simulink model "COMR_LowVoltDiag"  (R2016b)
settings: Solver=FixedStepDiscrete  StartTime=0.0  StopTime=10.0  FixedStep=1  RelTol=1e-3  EnableMultiTasking=on
undefined symbols (not defined in the file or in its folder): COMR_tiCSCPwrSpy_C, COMR_tiKl30cLowErr_C, COMR_tiKl30HighLowErr_C, COMR_tiKl30OurRang_C, COMR_uCSCVoltHiErr_C, COMR_uCSCVoltLoErr_C, COMR_uKl30cLowErrHeal_C, COMR_uKl30cLowErrHVOn_C, COMR_uKl30cLowErrNoHVOn_C, COMR_uKl30VlotHiErr_C, COMR_uKl30VlotHiHeal_C, COMR_uKl30VoltLoErr_C, COMR_uKl30VoltLoHeal_C, COMR_uKl30VoltOutRngHi_C, COMR_uKl30VoltOutRngLo_C
libraries: simulink x37

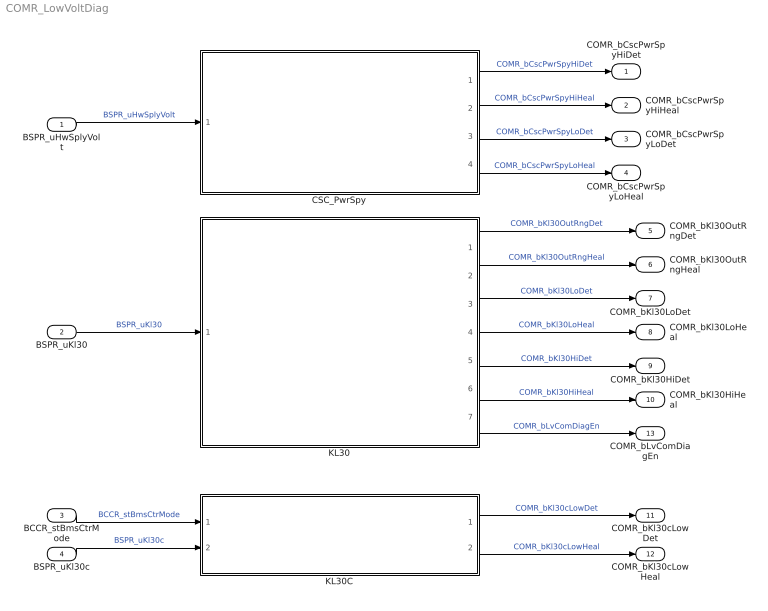
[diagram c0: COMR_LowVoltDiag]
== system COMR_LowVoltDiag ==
  BSPR_uHwSplyVolt : Inport
  BSPR_uKl30 : Inport  Port=2
  BCCR_stBmsCtrMode : Inport  Port=3
  BSPR_uKl30c : Inport  Port=4
  CSC_PwrSpy : Subsystem
  KL30 : Subsystem
  KL30C : Subsystem
  COMR_bCscPwrSpyHiDet : Outport
  COMR_bCscPwrSpyHiHeal : Outport  Port=2
  COMR_bCscPwrSpyLoDet : Outport  Port=3
  COMR_bCscPwrSpyLoHeal : Outport  Port=4
  COMR_bKl30OutRngDet : Outport  Port=5
  COMR_bKl30OutRngHeal : Outport  Port=6
  COMR_bKl30LoDet : Outport  Port=7
  COMR_bKl30LoHeal : Outport  Port=8
  COMR_bKl30HiDet : Outport  Port=9
  COMR_bKl30HiHeal : Outport  Port=10
  COMR_bKl30cLowDet : Outport  Port=11
  COMR_bKl30cLowHeal : Outport  Port=12
  COMR_bLvComDiagEn : Outport  Port=13
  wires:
  BSPR_uHwSplyVolt/1 -> CSC_PwrSpy/1(BSPR_uHwSplyVolt)  "BSPR_uHwSplyVolt"
  BSPR_uKl30/1 -> KL30/1(BSPR_uKl30)  "BSPR_uKl30"
  BCCR_stBmsCtrMode/1 -> KL30C/1(BCCR_stBmsCtrMode)  "BCCR_stBmsCtrMode"
  BSPR_uKl30c/1 -> KL30C/2(BSPR_uKl30c)  "BSPR_uKl30c"
  CSC_PwrSpy/4(COMR_bCscPwrSpyLoHeal) -> COMR_bCscPwrSpyLoHeal/1  "COMR_bCscPwrSpyLoHeal"
  CSC_PwrSpy/1(COMR_bCscPwrSpyHiDet) -> COMR_bCscPwrSpyHiDet/1  "COMR_bCscPwrSpyHiDet"
  CSC_PwrSpy/2(COMR_bCscPwrSpyHiHeal) -> COMR_bCscPwrSpyHiHeal/1  "COMR_bCscPwrSpyHiHeal"
  CSC_PwrSpy/3(COMR_bCscPwrSpyLoDet) -> COMR_bCscPwrSpyLoDet/1  "COMR_bCscPwrSpyLoDet"
  KL30/1(COMR_bKl30OutRngDet) -> COMR_bKl30OutRngDet/1  "COMR_bKl30OutRngDet"
  KL30/2(COMR_bKl30OutRngHeal) -> COMR_bKl30OutRngHeal/1  "COMR_bKl30OutRngHeal"
  KL30/3(COMR_bKl30LoDet) -> COMR_bKl30LoDet/1  "COMR_bKl30LoDet"
  KL30/5(COMR_bKl30HiDet) -> COMR_bKl30HiDet/1  "COMR_bKl30HiDet"
  KL30/4(COMR_bKl30LoHeal) -> COMR_bKl30LoHeal/1  "COMR_bKl30LoHeal"
  KL30/6(COMR_bKl30HiHeal) -> COMR_bKl30HiHeal/1  "COMR_bKl30HiHeal"
  KL30C/1(COMR_bKl30cLowDet) -> COMR_bKl30cLowDet/1  "COMR_bKl30cLowDet"
  KL30C/2(COMR_bKl30cLowHeal) -> COMR_bKl30cLowHeal/1  "COMR_bKl30cLowHeal"
  KL30/7(COMR_bLvComDiagEn) -> COMR_bLvComDiagEn/1  "COMR_bLvComDiagEn"

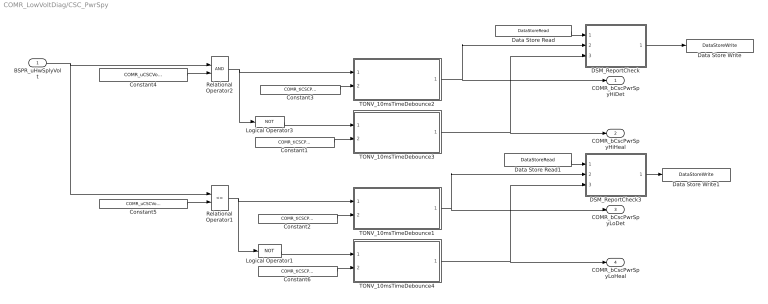
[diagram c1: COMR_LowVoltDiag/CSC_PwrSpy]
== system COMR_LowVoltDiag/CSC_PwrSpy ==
  BSPR_uHwSplyVolt : Inport
  Constant{1..3,6} (4 alike) : Constant  Value=COMR_tiCSCPwrSpy_C
  Constant4 : Constant  Value=COMR_uCSCVoltHiErr_C
  Constant5 : Constant  Value=COMR_uCSCVoltLoErr_C
  DSM_ReportCheck : Subsystem  TreatAsAtomicUnit=on  RTWFcnName=DSM_ReportCheck  RTWFileName=SrvLib
  DSM_ReportCheck3 : Subsystem  TreatAsAtomicUnit=on  RTWFcnName=DSM_ReportCheck  RTWFileName=SrvLib
  Data Store Read : DataStoreRead  DataStoreName=DFC_CSCPwrSpyHiErr
  Data Store Read1 : DataStoreRead  DataStoreName=DFC_CSCPwrSpyLoErr
  Data Store Write : DataStoreWrite  DataStoreName=DFC_CSCPwrSpyHiErr
  Data Store Write1 : DataStoreWrite  DataStoreName=DFC_CSCPwrSpyLoErr
  Logical Operator1 : Logic  Operator=NOT  AllPortsSameDT=off  OutDataTypeStr=boolean
  Logical Operator3 : Logic  Operator=NOT  AllPortsSameDT=off  OutDataTypeStr=boolean
  Relational Operator1 : RelationalOperator  Operator=<=  OutDataTypeStr=boolean  RndMeth=Simplest
  Relational Operator2 : RelationalOperator  OutDataTypeStr=boolean  RndMeth=Simplest
  TONV_10msTimeDebounce1 : Subsystem  TreatAsAtomicUnit=on  RTWFcnName=TONV_10msTimeDebounce  RTWFileName=SrvLib
  TONV_10msTimeDebounce2 : Subsystem  TreatAsAtomicUnit=on  RTWFcnName=TONV_10msTimeDebounce  RTWFileName=SrvLib
  TONV_10msTimeDebounce3 : Subsystem  TreatAsAtomicUnit=on  RTWFcnName=TONV_10msTimeDebounce  RTWFileName=SrvLib
  TONV_10msTimeDebounce4 : Subsystem  TreatAsAtomicUnit=on  RTWFcnName=TONV_10msTimeDebounce  RTWFileName=SrvLib
  COMR_bCscPwrSpyHiDet : Outport
  COMR_bCscPwrSpyHiHeal : Outport  Port=2
  COMR_bCscPwrSpyLoDet : Outport  Port=3
  COMR_bCscPwrSpyLoHeal : Outport  Port=4
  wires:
  Constant4/1 -> Relational Operator2/2
  BSPR_uHwSplyVolt/1 -> Relational Operator2/1, Relational Operator1/1
  TONV_10msTimeDebounce2/1(y) -> DSM_ReportCheck/2(Err), COMR_bCscPwrSpyHiDet/1
  Relational Operator2/1 -> TONV_10msTimeDebounce2/1(u), Logical Operator3/1
  DSM_ReportCheck/1(Dfc_id) -> Data Store Write/1
  Constant3/1 -> TONV_10msTimeDebounce2/2(T)
  Constant2/1 -> TONV_10msTimeDebounce1/2(T)
  Relational Operator1/1 -> Logical Operator1/1, TONV_10msTimeDebounce1/1(u)
  TONV_10msTimeDebounce1/1(y) -> DSM_ReportCheck3/2(Err), COMR_bCscPwrSpyLoDet/1
  DSM_ReportCheck3/1(Dfc_id) -> Data Store Write1/1
  Constant5/1 -> Relational Operator1/2
  Logical Operator3/1 -> TONV_10msTimeDebounce3/1(u)
  Constant1/1 -> TONV_10msTimeDebounce3/2(T)
  TONV_10msTimeDebounce3/1(y) -> DSM_ReportCheck/3(Heal), COMR_bCscPwrSpyHiHeal/1
  Data Store Read/1 -> DSM_ReportCheck/1(Dfc_id_nv)
  Logical Operator1/1 -> TONV_10msTimeDebounce4/1(u)
  Constant6/1 -> TONV_10msTimeDebounce4/2(T)
  TONV_10msTimeDebounce4/1(y) -> DSM_ReportCheck3/3(Heal), COMR_bCscPwrSpyLoHeal/1
  Data Store Read1/1 -> DSM_ReportCheck3/1(Dfc_id_nv)

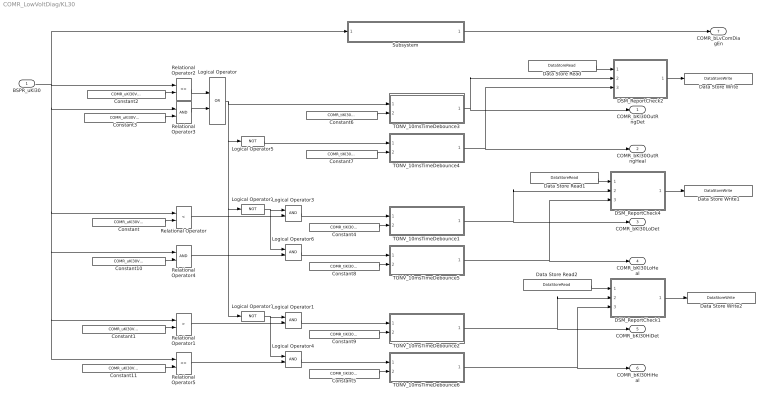
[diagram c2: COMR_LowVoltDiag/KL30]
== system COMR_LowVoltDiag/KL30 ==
  BSPR_uKl30 : Inport
  Constant : Constant  Value=COMR_uKl30VoltLoErr_C
  Constant1 : Constant  Value=COMR_uKl30VlotHiErr_C
  Constant10 : Constant  Value=COMR_uKl30VoltLoHeal_C
  Constant11 : Constant  Value=COMR_uKl30VlotHiHeal_C
  Constant2 : Constant  Value=COMR_uKl30VoltOutRngLo_C
  Constant3 : Constant  Value=COMR_uKl30VoltOutRngHi_C
  Constant{4..5,8..9} (4 alike) : Constant  Value=COMR_tiKl30HighLowErr_C
  Constant6 : Constant  Value=COMR_tiKl30OurRang_C
  Constant7 : Constant  Value=COMR_tiKl30OurRang_C
  DSM_ReportCheck1 : Subsystem  TreatAsAtomicUnit=on  RTWFcnName=DSM_ReportCheck  RTWFileName=SrvLib
  DSM_ReportCheck2 : Subsystem  TreatAsAtomicUnit=on  RTWFcnName=DSM_ReportCheck  RTWFileName=SrvLib
  DSM_ReportCheck4 : Subsystem  TreatAsAtomicUnit=on  RTWFcnName=DSM_ReportCheck  RTWFileName=SrvLib
  Data Store Read : DataStoreRead  DataStoreName=DFC_Kl30OutRngErr
  Data Store Read1 : DataStoreRead  DataStoreName=DFC_Kl30VoltLoErr
  Data Store Read2 : DataStoreRead  DataStoreName=DFC_Kl30VoltHiErr
  Data Store Write : DataStoreWrite  DataStoreName=DFC_Kl30OutRngErr
  Data Store Write1 : DataStoreWrite  DataStoreName=DFC_Kl30VoltLoErr
  Data Store Write2 : DataStoreWrite  DataStoreName=DFC_Kl30VoltHiErr
  Logical Operator : Logic  Operator=OR  AllPortsSameDT=off  OutDataTypeStr=boolean
  Logical Operator{1,3..4,6} (4 alike) : Logic  AllPortsSameDT=off  OutDataTypeStr=boolean
  Logical Operator2 : Logic  Operator=NOT  AllPortsSameDT=off  OutDataTypeStr=boolean
  Logical Operator5 : Logic  Operator=NOT  AllPortsSameDT=off  OutDataTypeStr=boolean
  Logical Operator7 : Logic  Operator=NOT  AllPortsSameDT=off  OutDataTypeStr=boolean
  Relational Operator : RelationalOperator  Operator=<  OutDataTypeStr=boolean  RndMeth=Simplest
  Relational Operator1 : RelationalOperator  Operator=>  OutDataTypeStr=boolean  RndMeth=Simplest
  Relational Operator2 : RelationalOperator  Operator=<=  OutDataTypeStr=boolean  RndMeth=Simplest
  Relational Operator3 : RelationalOperator  OutDataTypeStr=boolean  RndMeth=Simplest
  Relational Operator4 : RelationalOperator  OutDataTypeStr=boolean  RndMeth=Simplest
  Relational Operator5 : RelationalOperator  Operator=<=  OutDataTypeStr=boolean  RndMeth=Simplest
  Subsystem : Subsystem
  TONV_10msTimeDebounce1 : Subsystem  TreatAsAtomicUnit=on  RTWFcnName=TONV_10msTimeDebounce  RTWFileName=SrvLib
  TONV_10msTimeDebounce2 : Subsystem  TreatAsAtomicUnit=on  RTWFcnName=TONV_10msTimeDebounce  RTWFileName=SrvLib
  TONV_10msTimeDebounce3 : Subsystem  TreatAsAtomicUnit=on  RTWFcnName=TONV_10msTimeDebounce  RTWFileName=SrvLib
  TONV_10msTimeDebounce4 : Subsystem  TreatAsAtomicUnit=on  RTWFcnName=TONV_10msTimeDebounce  RTWFileName=SrvLib
  TONV_10msTimeDebounce5 : Subsystem  TreatAsAtomicUnit=on  RTWFcnName=TONV_10msTimeDebounce  RTWFileName=SrvLib
  TONV_10msTimeDebounce6 : Subsystem  TreatAsAtomicUnit=on  RTWFcnName=TONV_10msTimeDebounce  RTWFileName=SrvLib
  COMR_bKl30OutRngDet : Outport
  COMR_bKl30OutRngHeal : Outport  Port=2
  COMR_bKl30LoDet : Outport  Port=3
  COMR_bKl30LoHeal : Outport  Port=4
  COMR_bKl30HiDet : Outport  Port=5
  COMR_bKl30HiHeal : Outport  Port=6
  COMR_bLvComDiagEn : Outport  Port=7
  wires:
  Constant5/1 -> TONV_10msTimeDebounce6/2(T)
  TONV_10msTimeDebounce6/1(y) -> COMR_bKl30HiHeal/1, DSM_ReportCheck1/3(Heal)
  Data Store Read1/1 -> DSM_ReportCheck4/1(Dfc_id_nv)
  Data Store Read2/1 -> DSM_ReportCheck1/1(Dfc_id_nv)
  Logical Operator3/1 -> TONV_10msTimeDebounce1/1(u)
  Constant9/1 -> TONV_10msTimeDebounce2/2(T)
  Constant4/1 -> TONV_10msTimeDebounce1/2(T)
  Relational Operator3/1 -> Logical Operator/2
  Relational Operator2/1 -> Logical Operator/1
  TONV_10msTimeDebounce1/1(y) -> DSM_ReportCheck4/2(Err), COMR_bKl30LoDet/1
  Constant7/1 -> TONV_10msTimeDebounce4/2(T)
  Data Store Read/1 -> DSM_ReportCheck2/1(Dfc_id_nv)
  TONV_10msTimeDebounce2/1(y) -> DSM_ReportCheck1/2(Err), COMR_bKl30HiDet/1
  DSM_ReportCheck1/1(Dfc_id) -> Data Store Write2/1
  TONV_10msTimeDebounce3/1(y) -> COMR_bKl30OutRngDet/1, DSM_ReportCheck2/2(Err)
  DSM_ReportCheck2/1(Dfc_id) -> Data Store Write/1
  Constant6/1 -> TONV_10msTimeDebounce3/2(T)
  Logical Operator5/1 -> TONV_10msTimeDebounce4/1(u)
  DSM_ReportCheck4/1(Dfc_id) -> Data Store Write1/1
  TONV_10msTimeDebounce4/1(y) -> COMR_bKl30OutRngHeal/1, DSM_ReportCheck2/3(Heal)
  Logical Operator/1 -> Logical Operator7/1, Logical Operator2/1, Logical Operator5/1, TONV_10msTimeDebounce3/1(u)
  Logical Operator1/1 -> TONV_10msTimeDebounce2/1(u)
  Constant3/1 -> Relational Operator3/2
  Constant2/1 -> Relational Operator2/2
  TONV_10msTimeDebounce5/1(y) -> COMR_bKl30LoHeal/1, DSM_ReportCheck4/3(Heal)
  Constant8/1 -> TONV_10msTimeDebounce5/2(T)
  Relational Operator4/1 -> Logical Operator6/2
  Relational Operator1/1 -> Logical Operator1/2
  Constant1/1 -> Relational Operator1/2
  Constant/1 -> Relational Operator/2
  BSPR_uKl30/1 -> Relational Operator2/1, Relational Operator3/1, Relational Operator/1, Relational Operator4/1, Relational Operator5/1, Relational Operator1/1, Subsystem/1(BSPR_uKl30)
  Relational Operator/1 -> Logical Operator3/2
  Logical Operator2/1 -> Logical Operator6/1, Logical Operator3/1
  Logical Operator7/1 -> Logical Operator4/1, Logical Operator1/1
  Subsystem/1(COMR_bLvComDiagEn) -> COMR_bLvComDiagEn/1
  Constant10/1 -> Relational Operator4/2
  Constant11/1 -> Relational Operator5/2
  Relational Operator5/1 -> Logical Operator4/2
  Logical Operator4/1 -> TONV_10msTimeDebounce6/1(u)
  Logical Operator6/1 -> TONV_10msTimeDebounce5/1(u)

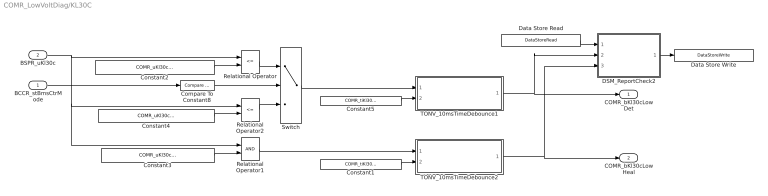
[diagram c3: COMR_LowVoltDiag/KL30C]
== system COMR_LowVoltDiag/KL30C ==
  BCCR_stBmsCtrMode : Inport
  BSPR_uKl30c : Inport  Port=2
  Compare To Constant8 : simulink/Logic and Bit Operations/Compare To Constant  relop===  const=4  OutDataTypeStr=boolean
  Constant1 : Constant  Value=COMR_tiKl30cLowErr_C  OutDataTypeStr=single
  Constant2 : Constant  Value=COMR_uKl30cLowErrHVOn_C  OutDataTypeStr=single
  Constant3 : Constant  Value=COMR_uKl30cLowErrHeal_C  OutDataTypeStr=single
  Constant4 : Constant  Value=COMR_uKl30cLowErrNoHVOn_C  OutDataTypeStr=single
  Constant5 : Constant  Value=COMR_tiKl30cLowErr_C  OutDataTypeStr=single
  DSM_ReportCheck2 : Subsystem  TreatAsAtomicUnit=on  RTWFcnName=DSM_ReportCheck  RTWFileName=SrvLib
  Data Store Read : DataStoreRead  DataStoreName=DFC_Kl30cVoltLoErr
  Data Store Write : DataStoreWrite  DataStoreName=DFC_Kl30cVoltLoErr
  Relational Operator : RelationalOperator  Operator=<=  OutDataTypeStr=boolean  RndMeth=Simplest
  Relational Operator1 : RelationalOperator  OutDataTypeStr=boolean  RndMeth=Simplest
  Relational Operator2 : RelationalOperator  Operator=<=  OutDataTypeStr=boolean  RndMeth=Simplest
  Switch : Switch  Criteria=u2 > Threshold
  TONV_10msTimeDebounce1 : Subsystem  TreatAsAtomicUnit=on  RTWFcnName=TONV_10msTimeDebounce  RTWFileName=SrvLib
  TONV_10msTimeDebounce2 : Subsystem  TreatAsAtomicUnit=on  RTWFcnName=TONV_10msTimeDebounce  RTWFileName=SrvLib
  COMR_bKl30cLowDet : Outport
  COMR_bKl30cLowHeal : Outport  Port=2
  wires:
  Constant1/1 -> TONV_10msTimeDebounce2/2(T)
  Data Store Read/1 -> DSM_ReportCheck2/1(Dfc_id_nv)
  Constant2/1 -> Relational Operator/2
  BSPR_uKl30c/1 -> Relational Operator/1, Relational Operator2/1, Relational Operator1/1
  Relational Operator/1 -> Switch/1
  Constant5/1 -> TONV_10msTimeDebounce1/2(T)
  Relational Operator2/1 -> Switch/3
  TONV_10msTimeDebounce2/1(y) -> COMR_bKl30cLowHeal/1, DSM_ReportCheck2/3(Heal)
  TONV_10msTimeDebounce1/1(y) -> DSM_ReportCheck2/2(Err), COMR_bKl30cLowDet/1
  Compare To Constant8/1 -> Switch/2
  Constant4/1 -> Relational Operator2/2
  BCCR_stBmsCtrMode/1 -> Compare To Constant8/1
  DSM_ReportCheck2/1(Dfc_id) -> Data Store Write/1
  Switch/1 -> TONV_10msTimeDebounce1/1(u)
  Relational Operator1/1 -> TONV_10msTimeDebounce2/1(u)
  Constant3/1 -> Relational Operator1/2

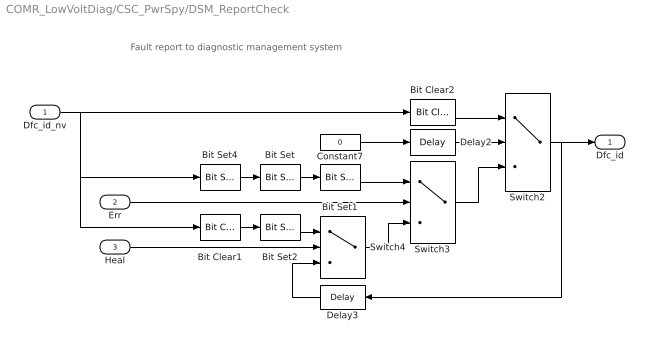
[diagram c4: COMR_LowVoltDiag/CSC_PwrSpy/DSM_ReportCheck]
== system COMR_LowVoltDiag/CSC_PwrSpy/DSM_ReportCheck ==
  note: Fault report to diagnostic management system
  Dfc_id_nv : Inport  OutDataTypeStr=uint8
  Err : Inport  Port=2
  Heal : Inport  Port=3
  Bit Clear1 : simulink/Logic and Bit Operations/Bit Clear  iBit=4
  Bit Clear2 : simulink/Logic and Bit Operations/Bit Clear  iBit=3
  Bit Set : simulink/Logic and Bit Operations/Bit Set  iBit=4
  Bit Set1 : simulink/Logic and Bit Operations/Bit Set  iBit=3
  Bit Set2 : simulink/Logic and Bit Operations/Bit Set  iBit=3
  Bit Set4 : simulink/Logic and Bit Operations/Bit Set  iBit=7
  Constant7 : Constant  Value=0  OutDataTypeStr=boolean
  Delay2 : Delay  DelayLength=1  InitialCondition=1
  Delay3 : Delay  DelayLength=1  InitialCondition=0
  Switch2 : Switch  Criteria=u2 ~= 0
  Switch3 : Switch  Criteria=u2 ~= 0
  Switch4 : Switch  Criteria=u2 ~= 0
  Dfc_id : Outport  OutDataTypeStr=uint8
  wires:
  Dfc_id_nv/1 -> Bit Clear2/1, Bit Set4/1, Bit Clear1/1
  Bit Set4/1 -> Bit Set/1
  Constant7/1 -> Delay2/1
  Delay2/1 -> Switch2/2
  Switch3/1 -> Switch2/3
  Bit Clear2/1 -> Switch2/1
  Switch2/1 -> Delay3/1, Dfc_id/1
  Bit Set1/1 -> Switch3/1
  Bit Set/1 -> Bit Set1/1
  Switch4/1 -> Switch3/3
  Err/1 -> Switch3/2
  Bit Set2/1 -> Switch4/1
  Bit Clear1/1 -> Bit Set2/1
  Delay3/1 -> Switch4/3
  Heal/1 -> Switch4/2

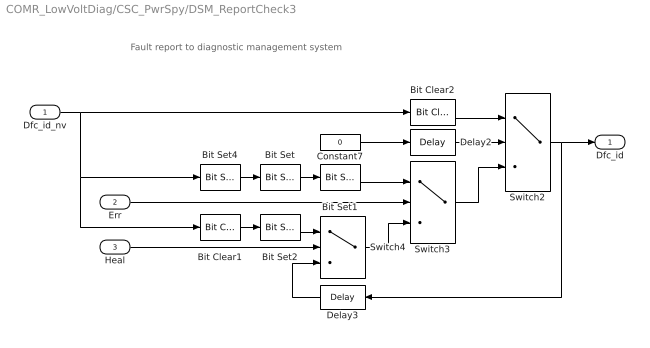
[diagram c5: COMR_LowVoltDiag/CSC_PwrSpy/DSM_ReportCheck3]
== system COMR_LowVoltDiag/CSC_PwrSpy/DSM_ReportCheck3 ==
  note: Fault report to diagnostic management system
  Dfc_id_nv : Inport  OutDataTypeStr=uint8
  Err : Inport  Port=2
  Heal : Inport  Port=3
  Bit Clear1 : simulink/Logic and Bit Operations/Bit Clear  iBit=4
  Bit Clear2 : simulink/Logic and Bit Operations/Bit Clear  iBit=3
  Bit Set : simulink/Logic and Bit Operations/Bit Set  iBit=4
  Bit Set1 : simulink/Logic and Bit Operations/Bit Set  iBit=3
  Bit Set2 : simulink/Logic and Bit Operations/Bit Set  iBit=3
  Bit Set4 : simulink/Logic and Bit Operations/Bit Set  iBit=7
  Constant7 : Constant  Value=0  OutDataTypeStr=boolean
  Delay2 : Delay  DelayLength=1  InitialCondition=1
  Delay3 : Delay  DelayLength=1  InitialCondition=0
  Switch2 : Switch  Criteria=u2 ~= 0
  Switch3 : Switch  Criteria=u2 ~= 0
  Switch4 : Switch  Criteria=u2 ~= 0
  Dfc_id : Outport  OutDataTypeStr=uint8
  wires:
  Dfc_id_nv/1 -> Bit Clear2/1, Bit Set4/1, Bit Clear1/1
  Bit Set4/1 -> Bit Set/1
  Constant7/1 -> Delay2/1
  Delay2/1 -> Switch2/2
  Switch3/1 -> Switch2/3
  Bit Clear2/1 -> Switch2/1
  Switch2/1 -> Delay3/1, Dfc_id/1
  Bit Set1/1 -> Switch3/1
  Bit Set/1 -> Bit Set1/1
  Switch4/1 -> Switch3/3
  Err/1 -> Switch3/2
  Bit Set2/1 -> Switch4/1
  Bit Clear1/1 -> Bit Set2/1
  Delay3/1 -> Switch4/3
  Heal/1 -> Switch4/2

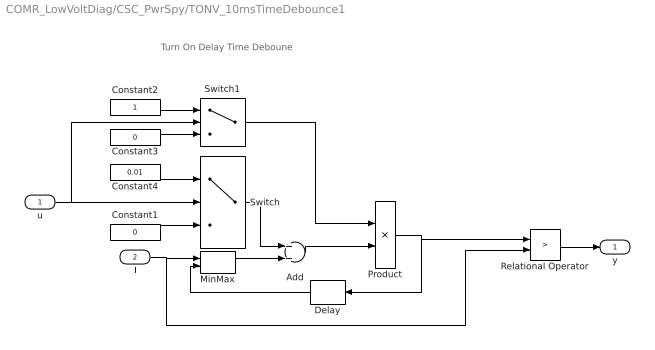
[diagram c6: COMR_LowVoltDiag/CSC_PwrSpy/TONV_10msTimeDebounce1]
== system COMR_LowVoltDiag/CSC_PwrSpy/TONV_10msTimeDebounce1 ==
  note: Turn On Delay Time Deboune
  u : Inport
  T : Inport  Port=2
  Add : Sum
  Constant1 : Constant  Value=0  OutDataTypeStr=single
  Constant2 : Constant  OutDataTypeStr=uint8
  Constant3 : Constant  Value=0  OutDataTypeStr=uint8
  Constant4 : Constant  Value=0.01  OutDataTypeStr=single
  Delay : Delay  DelayLength=1  InitialCondition=0
  MinMax : MinMax  Inputs=2
  Product : Product  OutMin=[0]  OutMax=[65535]  OutDataTypeStr=single
  Relational Operator : RelationalOperator  Operator=>  OutDataTypeStr=boolean  RndMeth=Simplest
  Switch : Switch  Criteria=u2 ~= 0
  Switch1 : Switch  Criteria=u2 ~= 0
  y : Outport
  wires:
  MinMax/1 -> Add/2
  T/1 -> Relational Operator/2, MinMax/1
  Relational Operator/1 -> y/1
  Delay/1 -> MinMax/2
  Switch/1 -> Add/1
  Product/1 -> Delay/1, Relational Operator/1
  Add/1 -> Product/2
  Constant1/1 -> Switch/3
  Constant4/1 -> Switch/1
  u/1 -> Switch/2, Switch1/2
  Constant2/1 -> Switch1/1
  Constant3/1 -> Switch1/3
  Switch1/1 -> Product/1

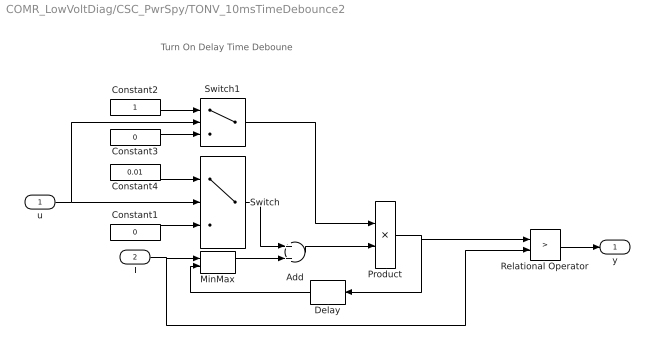
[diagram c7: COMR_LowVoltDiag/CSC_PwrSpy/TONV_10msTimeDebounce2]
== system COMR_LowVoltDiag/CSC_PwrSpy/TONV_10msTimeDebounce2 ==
  note: Turn On Delay Time Deboune
  u : Inport
  T : Inport  Port=2
  Add : Sum
  Constant1 : Constant  Value=0  OutDataTypeStr=single
  Constant2 : Constant  OutDataTypeStr=uint8
  Constant3 : Constant  Value=0  OutDataTypeStr=uint8
  Constant4 : Constant  Value=0.01  OutDataTypeStr=single
  Delay : Delay  DelayLength=1  InitialCondition=0
  MinMax : MinMax  Inputs=2
  Product : Product  OutMin=[0]  OutMax=[65535]  OutDataTypeStr=single
  Relational Operator : RelationalOperator  Operator=>  OutDataTypeStr=boolean  RndMeth=Simplest
  Switch : Switch  Criteria=u2 ~= 0
  Switch1 : Switch  Criteria=u2 ~= 0
  y : Outport
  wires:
  MinMax/1 -> Add/2
  T/1 -> Relational Operator/2, MinMax/1
  Relational Operator/1 -> y/1
  Delay/1 -> MinMax/2
  Switch/1 -> Add/1
  Product/1 -> Delay/1, Relational Operator/1
  Add/1 -> Product/2
  Constant1/1 -> Switch/3
  Constant4/1 -> Switch/1
  u/1 -> Switch/2, Switch1/2
  Constant2/1 -> Switch1/1
  Constant3/1 -> Switch1/3
  Switch1/1 -> Product/1

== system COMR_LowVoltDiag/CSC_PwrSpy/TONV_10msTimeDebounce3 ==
  note: Turn On Delay Time Deboune
  u : Inport
  T : Inport  Port=2
  Add : Sum
  Constant1 : Constant  Value=0  OutDataTypeStr=single
  Constant2 : Constant  OutDataTypeStr=uint8
  Constant3 : Constant  Value=0  OutDataTypeStr=uint8
  Constant4 : Constant  Value=0.01  OutDataTypeStr=single
  Delay : Delay  DelayLength=1  InitialCondition=0
  MinMax : MinMax  Inputs=2
  Product : Product  OutMin=[0]  OutMax=[65535]  OutDataTypeStr=single
  Relational Operator : RelationalOperator  Operator=>  OutDataTypeStr=boolean  RndMeth=Simplest
  Switch : Switch  Criteria=u2 ~= 0
  Switch1 : Switch  Criteria=u2 ~= 0
  y : Outport
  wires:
  MinMax/1 -> Add/2
  T/1 -> Relational Operator/2, MinMax/1
  Relational Operator/1 -> y/1
  Delay/1 -> MinMax/2
  Switch/1 -> Add/1
  Product/1 -> Delay/1, Relational Operator/1
  Add/1 -> Product/2
  Constant1/1 -> Switch/3
  Constant4/1 -> Switch/1
  u/1 -> Switch/2, Switch1/2
  Constant2/1 -> Switch1/1
  Constant3/1 -> Switch1/3
  Switch1/1 -> Product/1

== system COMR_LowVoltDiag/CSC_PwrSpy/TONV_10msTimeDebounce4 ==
  note: Turn On Delay Time Deboune
  u : Inport
  T : Inport  Port=2
  Add : Sum
  Constant1 : Constant  Value=0  OutDataTypeStr=single
  Constant2 : Constant  OutDataTypeStr=uint8
  Constant3 : Constant  Value=0  OutDataTypeStr=uint8
  Constant4 : Constant  Value=0.01  OutDataTypeStr=single
  Delay : Delay  DelayLength=1  InitialCondition=0
  MinMax : MinMax  Inputs=2
  Product : Product  OutMin=[0]  OutMax=[65535]  OutDataTypeStr=single
  Relational Operator : RelationalOperator  Operator=>  OutDataTypeStr=boolean  RndMeth=Simplest
  Switch : Switch  Criteria=u2 ~= 0
  Switch1 : Switch  Criteria=u2 ~= 0
  y : Outport
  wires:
  Switch1/1 -> Product/1
  Constant3/1 -> Switch1/3
  Constant2/1 -> Switch1/1
  u/1 -> Switch1/2, Switch/2
  Constant4/1 -> Switch/1
  Constant1/1 -> Switch/3
  Add/1 -> Product/2
  Product/1 -> Relational Operator/1, Delay/1
  Switch/1 -> Add/1
  Delay/1 -> MinMax/2
  Relational Operator/1 -> y/1
  T/1 -> MinMax/1, Relational Operator/2
  MinMax/1 -> Add/2

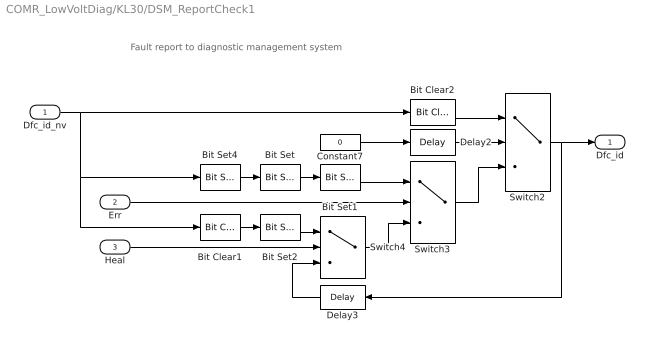
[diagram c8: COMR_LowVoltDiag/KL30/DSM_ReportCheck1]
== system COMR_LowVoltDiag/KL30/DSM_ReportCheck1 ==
  note: Fault report to diagnostic management system
  Dfc_id_nv : Inport  OutDataTypeStr=uint8
  Err : Inport  Port=2
  Heal : Inport  Port=3
  Bit Clear1 : simulink/Logic and Bit Operations/Bit Clear  iBit=4
  Bit Clear2 : simulink/Logic and Bit Operations/Bit Clear  iBit=3
  Bit Set : simulink/Logic and Bit Operations/Bit Set  iBit=4
  Bit Set1 : simulink/Logic and Bit Operations/Bit Set  iBit=3
  Bit Set2 : simulink/Logic and Bit Operations/Bit Set  iBit=3
  Bit Set4 : simulink/Logic and Bit Operations/Bit Set  iBit=7
  Constant7 : Constant  Value=0  OutDataTypeStr=boolean
  Delay2 : Delay  DelayLength=1  InitialCondition=1
  Delay3 : Delay  DelayLength=1  InitialCondition=0
  Switch2 : Switch  Criteria=u2 ~= 0
  Switch3 : Switch  Criteria=u2 ~= 0
  Switch4 : Switch  Criteria=u2 ~= 0
  Dfc_id : Outport  OutDataTypeStr=uint8
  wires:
  Dfc_id_nv/1 -> Bit Clear2/1, Bit Set4/1, Bit Clear1/1
  Bit Set4/1 -> Bit Set/1
  Constant7/1 -> Delay2/1
  Delay2/1 -> Switch2/2
  Switch3/1 -> Switch2/3
  Bit Clear2/1 -> Switch2/1
  Switch2/1 -> Delay3/1, Dfc_id/1
  Bit Set1/1 -> Switch3/1
  Bit Set/1 -> Bit Set1/1
  Switch4/1 -> Switch3/3
  Err/1 -> Switch3/2
  Bit Set2/1 -> Switch4/1
  Bit Clear1/1 -> Bit Set2/1
  Delay3/1 -> Switch4/3
  Heal/1 -> Switch4/2

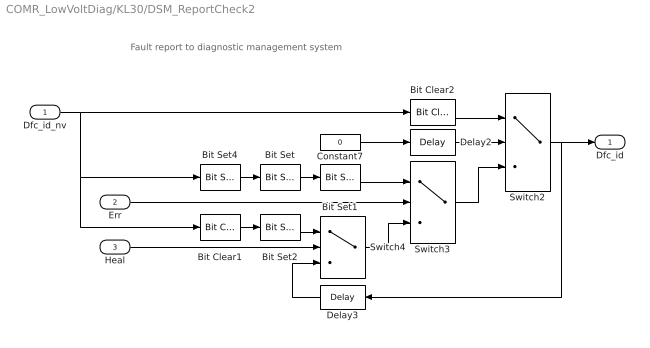
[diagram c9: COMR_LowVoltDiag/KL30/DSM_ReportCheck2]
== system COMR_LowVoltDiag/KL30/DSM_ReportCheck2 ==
  note: Fault report to diagnostic management system
  Dfc_id_nv : Inport  OutDataTypeStr=uint8
  Err : Inport  Port=2
  Heal : Inport  Port=3
  Bit Clear1 : simulink/Logic and Bit Operations/Bit Clear  iBit=4
  Bit Clear2 : simulink/Logic and Bit Operations/Bit Clear  iBit=3
  Bit Set : simulink/Logic and Bit Operations/Bit Set  iBit=4
  Bit Set1 : simulink/Logic and Bit Operations/Bit Set  iBit=3
  Bit Set2 : simulink/Logic and Bit Operations/Bit Set  iBit=3
  Bit Set4 : simulink/Logic and Bit Operations/Bit Set  iBit=7
  Constant7 : Constant  Value=0  OutDataTypeStr=boolean
  Delay2 : Delay  DelayLength=1  InitialCondition=1
  Delay3 : Delay  DelayLength=1  InitialCondition=0
  Switch2 : Switch  Criteria=u2 ~= 0
  Switch3 : Switch  Criteria=u2 ~= 0
  Switch4 : Switch  Criteria=u2 ~= 0
  Dfc_id : Outport  OutDataTypeStr=uint8
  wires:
  Dfc_id_nv/1 -> Bit Clear2/1, Bit Set4/1, Bit Clear1/1
  Bit Set4/1 -> Bit Set/1
  Constant7/1 -> Delay2/1
  Delay2/1 -> Switch2/2
  Switch3/1 -> Switch2/3
  Bit Clear2/1 -> Switch2/1
  Switch2/1 -> Delay3/1, Dfc_id/1
  Bit Set1/1 -> Switch3/1
  Bit Set/1 -> Bit Set1/1
  Switch4/1 -> Switch3/3
  Err/1 -> Switch3/2
  Bit Set2/1 -> Switch4/1
  Bit Clear1/1 -> Bit Set2/1
  Delay3/1 -> Switch4/3
  Heal/1 -> Switch4/2

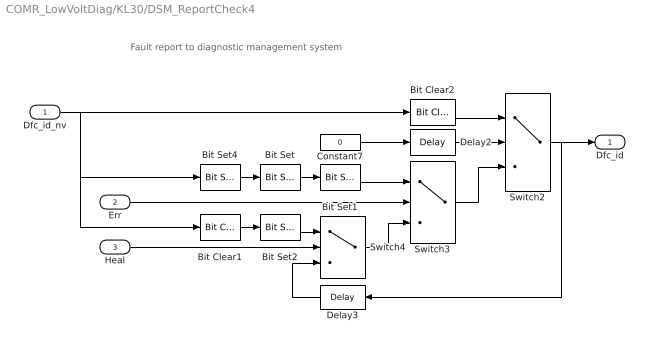
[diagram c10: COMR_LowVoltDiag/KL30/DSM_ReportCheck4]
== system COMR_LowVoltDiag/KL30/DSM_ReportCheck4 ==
  note: Fault report to diagnostic management system
  Dfc_id_nv : Inport  OutDataTypeStr=uint8
  Err : Inport  Port=2
  Heal : Inport  Port=3
  Bit Clear1 : simulink/Logic and Bit Operations/Bit Clear  iBit=4
  Bit Clear2 : simulink/Logic and Bit Operations/Bit Clear  iBit=3
  Bit Set : simulink/Logic and Bit Operations/Bit Set  iBit=4
  Bit Set1 : simulink/Logic and Bit Operations/Bit Set  iBit=3
  Bit Set2 : simulink/Logic and Bit Operations/Bit Set  iBit=3
  Bit Set4 : simulink/Logic and Bit Operations/Bit Set  iBit=7
  Constant7 : Constant  Value=0  OutDataTypeStr=boolean
  Delay2 : Delay  DelayLength=1  InitialCondition=1
  Delay3 : Delay  DelayLength=1  InitialCondition=0
  Switch2 : Switch  Criteria=u2 ~= 0
  Switch3 : Switch  Criteria=u2 ~= 0
  Switch4 : Switch  Criteria=u2 ~= 0
  Dfc_id : Outport  OutDataTypeStr=uint8
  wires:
  Dfc_id_nv/1 -> Bit Clear2/1, Bit Set4/1, Bit Clear1/1
  Bit Set4/1 -> Bit Set/1
  Constant7/1 -> Delay2/1
  Delay2/1 -> Switch2/2
  Switch3/1 -> Switch2/3
  Bit Clear2/1 -> Switch2/1
  Switch2/1 -> Delay3/1, Dfc_id/1
  Bit Set1/1 -> Switch3/1
  Bit Set/1 -> Bit Set1/1
  Switch4/1 -> Switch3/3
  Err/1 -> Switch3/2
  Bit Set2/1 -> Switch4/1
  Bit Clear1/1 -> Bit Set2/1
  Delay3/1 -> Switch4/3
  Heal/1 -> Switch4/2

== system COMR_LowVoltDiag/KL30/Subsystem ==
  BSPR_uKl30 : Inport
  ComDiagEn : Stateflow chart  TreatAsAtomicUnit=on
  COMR_bLvComDiagEn : Outport
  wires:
  ComDiagEn/1(COMR_bLvComDiagEn) -> COMR_bLvComDiagEn/1
  BSPR_uKl30/1 -> ComDiagEn/1(BSPR_uKl30)

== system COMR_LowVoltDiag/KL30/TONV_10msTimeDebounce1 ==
  note: Turn On Delay Time Deboune
  u : Inport
  T : Inport  Port=2
  Add : Sum
  Constant1 : Constant  Value=0  OutDataTypeStr=single
  Constant2 : Constant  OutDataTypeStr=uint8
  Constant3 : Constant  Value=0  OutDataTypeStr=uint8
  Constant4 : Constant  Value=0.01  OutDataTypeStr=single
  Delay : Delay  DelayLength=1  InitialCondition=0
  MinMax : MinMax  Inputs=2
  Product : Product  OutMin=[0]  OutMax=[65535]  OutDataTypeStr=single
  Relational Operator : RelationalOperator  Operator=>  OutDataTypeStr=boolean  RndMeth=Simplest
  Switch : Switch  Criteria=u2 ~= 0
  Switch1 : Switch  Criteria=u2 ~= 0
  y : Outport
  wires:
  MinMax/1 -> Add/2
  T/1 -> Relational Operator/2, MinMax/1
  Relational Operator/1 -> y/1
  Delay/1 -> MinMax/2
  Switch/1 -> Add/1
  Product/1 -> Delay/1, Relational Operator/1
  Add/1 -> Product/2
  Constant1/1 -> Switch/3
  Constant4/1 -> Switch/1
  u/1 -> Switch/2, Switch1/2
  Constant2/1 -> Switch1/1
  Constant3/1 -> Switch1/3
  Switch1/1 -> Product/1

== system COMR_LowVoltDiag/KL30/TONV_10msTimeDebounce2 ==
  note: Turn On Delay Time Deboune
  u : Inport
  T : Inport  Port=2
  Add : Sum
  Constant1 : Constant  Value=0  OutDataTypeStr=single
  Constant2 : Constant  OutDataTypeStr=uint8
  Constant3 : Constant  Value=0  OutDataTypeStr=uint8
  Constant4 : Constant  Value=0.01  OutDataTypeStr=single
  Delay : Delay  DelayLength=1  InitialCondition=0
  MinMax : MinMax  Inputs=2
  Product : Product  OutMin=[0]  OutMax=[65535]  OutDataTypeStr=single
  Relational Operator : RelationalOperator  Operator=>  OutDataTypeStr=boolean  RndMeth=Simplest
  Switch : Switch  Criteria=u2 ~= 0
  Switch1 : Switch  Criteria=u2 ~= 0
  y : Outport
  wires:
  MinMax/1 -> Add/2
  T/1 -> Relational Operator/2, MinMax/1
  Relational Operator/1 -> y/1
  Delay/1 -> MinMax/2
  Switch/1 -> Add/1
  Product/1 -> Delay/1, Relational Operator/1
  Add/1 -> Product/2
  Constant1/1 -> Switch/3
  Constant4/1 -> Switch/1
  u/1 -> Switch/2, Switch1/2
  Constant2/1 -> Switch1/1
  Constant3/1 -> Switch1/3
  Switch1/1 -> Product/1

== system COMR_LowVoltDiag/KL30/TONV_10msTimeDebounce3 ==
  note: Turn On Delay Time Deboune
  u : Inport
  T : Inport  Port=2
  Add : Sum
  Constant1 : Constant  Value=0  OutDataTypeStr=single
  Constant2 : Constant  OutDataTypeStr=uint8
  Constant3 : Constant  Value=0  OutDataTypeStr=uint8
  Constant4 : Constant  Value=0.01  OutDataTypeStr=single
  Delay : Delay  DelayLength=1  InitialCondition=0
  MinMax : MinMax  Inputs=2
  Product : Product  OutMin=[0]  OutMax=[65535]  OutDataTypeStr=single
  Relational Operator : RelationalOperator  Operator=>  OutDataTypeStr=boolean  RndMeth=Simplest
  Switch : Switch  Criteria=u2 ~= 0
  Switch1 : Switch  Criteria=u2 ~= 0
  y : Outport
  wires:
  MinMax/1 -> Add/2
  T/1 -> Relational Operator/2, MinMax/1
  Relational Operator/1 -> y/1
  Delay/1 -> MinMax/2
  Switch/1 -> Add/1
  Product/1 -> Delay/1, Relational Operator/1
  Add/1 -> Product/2
  Constant1/1 -> Switch/3
  Constant4/1 -> Switch/1
  u/1 -> Switch/2, Switch1/2
  Constant2/1 -> Switch1/1
  Constant3/1 -> Switch1/3
  Switch1/1 -> Product/1

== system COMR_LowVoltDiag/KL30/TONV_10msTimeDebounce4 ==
  note: Turn On Delay Time Deboune
  u : Inport
  T : Inport  Port=2
  Add : Sum
  Constant1 : Constant  Value=0  OutDataTypeStr=single
  Constant2 : Constant  OutDataTypeStr=uint8
  Constant3 : Constant  Value=0  OutDataTypeStr=uint8
  Constant4 : Constant  Value=0.01  OutDataTypeStr=single
  Delay : Delay  DelayLength=1  InitialCondition=0
  MinMax : MinMax  Inputs=2
  Product : Product  OutMin=[0]  OutMax=[65535]  OutDataTypeStr=single
  Relational Operator : RelationalOperator  Operator=>  OutDataTypeStr=boolean  RndMeth=Simplest
  Switch : Switch  Criteria=u2 ~= 0
  Switch1 : Switch  Criteria=u2 ~= 0
  y : Outport
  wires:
  MinMax/1 -> Add/2
  T/1 -> Relational Operator/2, MinMax/1
  Relational Operator/1 -> y/1
  Delay/1 -> MinMax/2
  Switch/1 -> Add/1
  Product/1 -> Delay/1, Relational Operator/1
  Add/1 -> Product/2
  Constant1/1 -> Switch/3
  Constant4/1 -> Switch/1
  u/1 -> Switch/2, Switch1/2
  Constant2/1 -> Switch1/1
  Constant3/1 -> Switch1/3
  Switch1/1 -> Product/1

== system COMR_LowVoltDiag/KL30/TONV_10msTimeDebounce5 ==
  note: Turn On Delay Time Deboune
  u : Inport
  T : Inport  Port=2
  Add : Sum
  Constant1 : Constant  Value=0  OutDataTypeStr=single
  Constant2 : Constant  OutDataTypeStr=uint8
  Constant3 : Constant  Value=0  OutDataTypeStr=uint8
  Constant4 : Constant  Value=0.01  OutDataTypeStr=single
  Delay : Delay  DelayLength=1  InitialCondition=0
  MinMax : MinMax  Inputs=2
  Product : Product  OutMin=[0]  OutMax=[65535]  OutDataTypeStr=single
  Relational Operator : RelationalOperator  Operator=>  OutDataTypeStr=boolean  RndMeth=Simplest
  Switch : Switch  Criteria=u2 ~= 0
  Switch1 : Switch  Criteria=u2 ~= 0
  y : Outport
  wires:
  MinMax/1 -> Add/2
  T/1 -> Relational Operator/2, MinMax/1
  Relational Operator/1 -> y/1
  Delay/1 -> MinMax/2
  Switch/1 -> Add/1
  Product/1 -> Delay/1, Relational Operator/1
  Add/1 -> Product/2
  Constant1/1 -> Switch/3
  Constant4/1 -> Switch/1
  u/1 -> Switch/2, Switch1/2
  Constant2/1 -> Switch1/1
  Constant3/1 -> Switch1/3
  Switch1/1 -> Product/1

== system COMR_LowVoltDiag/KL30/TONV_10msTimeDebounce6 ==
  note: Turn On Delay Time Deboune
  u : Inport
  T : Inport  Port=2
  Add : Sum
  Constant1 : Constant  Value=0  OutDataTypeStr=single
  Constant2 : Constant  OutDataTypeStr=uint8
  Constant3 : Constant  Value=0  OutDataTypeStr=uint8
  Constant4 : Constant  Value=0.01  OutDataTypeStr=single
  Delay : Delay  DelayLength=1  InitialCondition=0
  MinMax : MinMax  Inputs=2
  Product : Product  OutMin=[0]  OutMax=[65535]  OutDataTypeStr=single
  Relational Operator : RelationalOperator  Operator=>  OutDataTypeStr=boolean  RndMeth=Simplest
  Switch : Switch  Criteria=u2 ~= 0
  Switch1 : Switch  Criteria=u2 ~= 0
  y : Outport
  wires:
  MinMax/1 -> Add/2
  T/1 -> Relational Operator/2, MinMax/1
  Relational Operator/1 -> y/1
  Delay/1 -> MinMax/2
  Switch/1 -> Add/1
  Product/1 -> Delay/1, Relational Operator/1
  Add/1 -> Product/2
  Constant1/1 -> Switch/3
  Constant4/1 -> Switch/1
  u/1 -> Switch/2, Switch1/2
  Constant2/1 -> Switch1/1
  Constant3/1 -> Switch1/3
  Switch1/1 -> Product/1

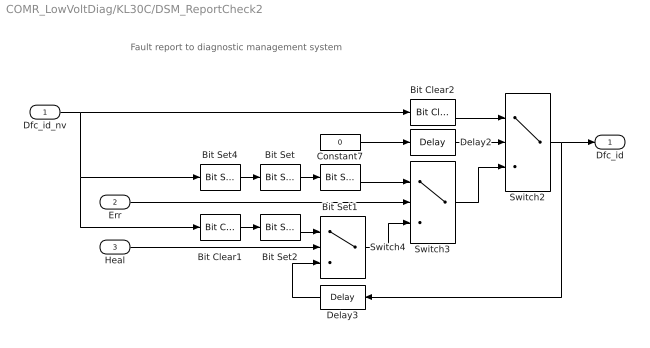
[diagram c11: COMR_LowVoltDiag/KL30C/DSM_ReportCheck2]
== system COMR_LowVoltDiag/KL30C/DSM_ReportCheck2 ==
  note: Fault report to diagnostic management system
  Dfc_id_nv : Inport  OutDataTypeStr=uint8
  Err : Inport  Port=2
  Heal : Inport  Port=3
  Bit Clear1 : simulink/Logic and Bit Operations/Bit Clear  iBit=4
  Bit Clear2 : simulink/Logic and Bit Operations/Bit Clear  iBit=3
  Bit Set : simulink/Logic and Bit Operations/Bit Set  iBit=4
  Bit Set1 : simulink/Logic and Bit Operations/Bit Set  iBit=3
  Bit Set2 : simulink/Logic and Bit Operations/Bit Set  iBit=3
  Bit Set4 : simulink/Logic and Bit Operations/Bit Set  iBit=7
  Constant7 : Constant  Value=0  OutDataTypeStr=boolean
  Delay2 : Delay  DelayLength=1  InitialCondition=1
  Delay3 : Delay  DelayLength=1  InitialCondition=0
  Switch2 : Switch  Criteria=u2 ~= 0
  Switch3 : Switch  Criteria=u2 ~= 0
  Switch4 : Switch  Criteria=u2 ~= 0
  Dfc_id : Outport  OutDataTypeStr=uint8
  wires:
  Dfc_id_nv/1 -> Bit Clear2/1, Bit Set4/1, Bit Clear1/1
  Bit Set4/1 -> Bit Set/1
  Constant7/1 -> Delay2/1
  Delay2/1 -> Switch2/2
  Switch3/1 -> Switch2/3
  Bit Clear2/1 -> Switch2/1
  Switch2/1 -> Delay3/1, Dfc_id/1
  Bit Set1/1 -> Switch3/1
  Bit Set/1 -> Bit Set1/1
  Switch4/1 -> Switch3/3
  Err/1 -> Switch3/2
  Bit Set2/1 -> Switch4/1
  Bit Clear1/1 -> Bit Set2/1
  Delay3/1 -> Switch4/3
  Heal/1 -> Switch4/2

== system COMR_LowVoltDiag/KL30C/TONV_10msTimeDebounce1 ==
  note: Turn On Delay Time Deboune
  u : Inport
  T : Inport  Port=2
  Add : Sum
  Constant1 : Constant  Value=0  OutDataTypeStr=single
  Constant2 : Constant  OutDataTypeStr=uint8
  Constant3 : Constant  Value=0  OutDataTypeStr=uint8
  Constant4 : Constant  Value=0.01  OutDataTypeStr=single
  Delay : Delay  DelayLength=1  InitialCondition=0
  MinMax : MinMax  Inputs=2
  Product : Product  OutMin=[0]  OutMax=[65535]  OutDataTypeStr=single
  Relational Operator : RelationalOperator  Operator=>  OutDataTypeStr=boolean  RndMeth=Simplest
  Switch : Switch  Criteria=u2 ~= 0
  Switch1 : Switch  Criteria=u2 ~= 0
  y : Outport
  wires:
  MinMax/1 -> Add/2
  T/1 -> Relational Operator/2, MinMax/1
  Relational Operator/1 -> y/1
  Delay/1 -> MinMax/2
  Switch/1 -> Add/1
  Product/1 -> Delay/1, Relational Operator/1
  Add/1 -> Product/2
  Constant1/1 -> Switch/3
  Constant4/1 -> Switch/1
  u/1 -> Switch/2, Switch1/2
  Constant2/1 -> Switch1/1
  Constant3/1 -> Switch1/3
  Switch1/1 -> Product/1

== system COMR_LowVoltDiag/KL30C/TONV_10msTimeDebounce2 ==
  note: Turn On Delay Time Deboune
  u : Inport
  T : Inport  Port=2
  Add : Sum
  Constant1 : Constant  Value=0  OutDataTypeStr=single
  Constant2 : Constant  OutDataTypeStr=uint8
  Constant3 : Constant  Value=0  OutDataTypeStr=uint8
  Constant4 : Constant  Value=0.01  OutDataTypeStr=single
  Delay : Delay  DelayLength=1  InitialCondition=0
  MinMax : MinMax  Inputs=2
  Product : Product  OutMin=[0]  OutMax=[65535]  OutDataTypeStr=single
  Relational Operator : RelationalOperator  Operator=>  OutDataTypeStr=boolean  RndMeth=Simplest
  Switch : Switch  Criteria=u2 ~= 0
  Switch1 : Switch  Criteria=u2 ~= 0
  y : Outport
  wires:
  MinMax/1 -> Add/2
  T/1 -> Relational Operator/2, MinMax/1
  Relational Operator/1 -> y/1
  Delay/1 -> MinMax/2
  Switch/1 -> Add/1
  Product/1 -> Delay/1, Relational Operator/1
  Add/1 -> Product/2
  Constant1/1 -> Switch/3
  Constant4/1 -> Switch/1
  u/1 -> Switch/2, Switch1/2
  Constant2/1 -> Switch1/1
  Constant3/1 -> Switch1/3
  Switch1/1 -> Product/1

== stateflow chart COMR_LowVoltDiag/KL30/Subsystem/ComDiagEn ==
  state Ini_Stt
    entry:
    counter = 0;
    COMR_bLvComDiagEn=boolean(0);
    during:
    counter = counter+0.01;
  state LowerDeb_Stt
    entry:
    counter = 0;
    COMR_bLvComDiagEn = boolean(0);
    during:
    counter = counter+0.01;
  state Normal_Stt
    entry:
    counter = 0;
    COMR_bLvComDiagEn = boolean(0);
    during:
    counter = counter+0.01;
  state Lower_Stt
    entry:
    counter = 0;
    COMR_bLvComDiagEn = boolean(0);
  state En_Stt
    entry:
    counter = 0;
    COMR_bLvComDiagEn=boolean(1);
  (default) -> Ini_Stt
  Ini_Stt -> Lower_Stt : [(BSPR_uKl30 < 9 || BSPR_uKl30 > 16) &&... counter >=0.05 ]
  Ini_Stt -> Normal_Stt : [BSPR_uKl30 >= 9 &&... BSPR_uKl30 <= 16 &&... counter >=0.05]
  Lower_Stt -> LowerDeb_Stt : [BSPR_uKl30 >= 10 &&... BSPR_uKl30 <= 15]
  Normal_Stt -> Lower_Stt : [BSPR_uKl30 < 9 ||... BSPR_uKl30 > 16]
  LowerDeb_Stt -> En_Stt : [counter>=2]
  Normal_Stt -> En_Stt : [counter>=2]
  En_Stt -> Lower_Stt : [BSPR_uKl30 < 9 || BSPR_uKl30 > 16]
  data: BSPR_uKl30 input single; COMR_bLvComDiagEn output boolean; counter local single
